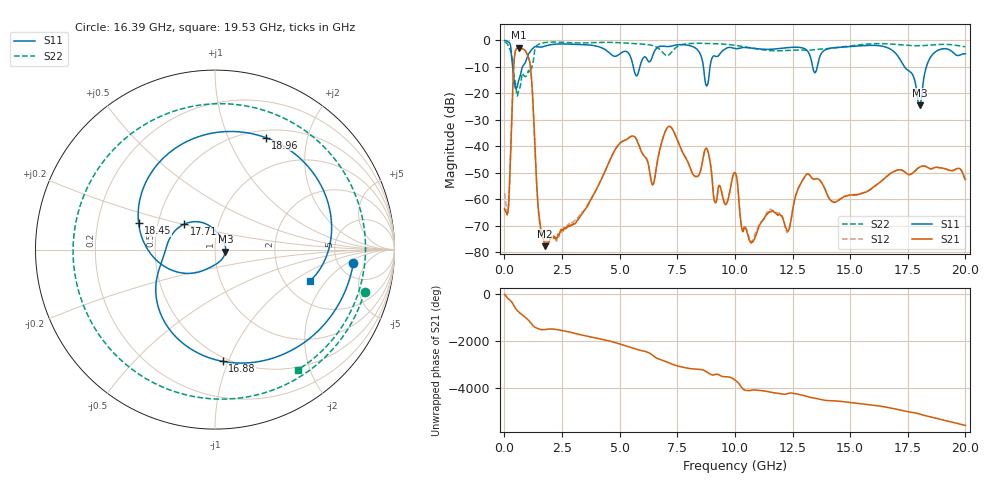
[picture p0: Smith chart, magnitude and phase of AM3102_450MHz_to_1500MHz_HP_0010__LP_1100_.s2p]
!Agilent Technologies,E8364B,MY43040894,A.07.50.67
!Agilent E8364B: A.07.50.67
!Date: Thursday, January 11, 2018 05:28:41
!Correction: S11(Full 2 Port(1,2))
!S21(Full 2 Port(1,2))
!S12(Full 2 Port(1,2))
!S22(Full 2 Port(1,2))
!S2P File: Measurements: S11, S21, S12, S22:
# Hz S  dB  R 50
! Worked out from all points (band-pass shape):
!   1601 points, 10 MHz to 20 GHz, reference 50 ohm
!   highest |S21| = -2.82 dB at 622.2 MHz (marker M1); lowest = -77.6 dB at 1.759 GHz (marker M2)
!   |S21| within 3 dB of the highest: 444.3 MHz to 1.018 GHz (573.5 MHz wide, 78.5 % of centre)
!   lowest |S11| = -24.6 dB at 18.01 GHz (marker M3), VSWR 1.13, Z = 56.2 - j1.29 ohm
!   |S11| at or under -10 dB: 356.9 MHz to 784 MHz (427.1 MHz wide, 74.9 % of centre); 5.593 GHz to 5.878 GHz (285.1 MHz wide, 4.97 % of centre); 17.35 GHz to 18.31 GHz (952.9 MHz wide, 5.34 % of centre)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
!   |S22| runs from -21.0 to -0.5 dB; largest |S21 - S12| = 0.0029
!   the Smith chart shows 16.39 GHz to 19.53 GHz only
!   S11 on the Smith chart (normalised r, x): 16.39 GHz: 6.94, -2.54; 16.88 GHz: 0.47, -0.95; 17.71 GHz: 0.68, +0.20; 18.45 GHz: 0.39, +0.14; 18.96 GHz: 0.59, +1.38; 19.53 GHz: 2.76, -1.39
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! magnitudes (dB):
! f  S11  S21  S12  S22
! 10 MHz  -0.1  -63.5  -57.6  -0.5
! 172.4 MHz  -0.6  -63.2  -63.4  -2.1
! 422.3 MHz  -15.3  -7.8  -7.8  -13.3
! 622.2 MHz  -15.1  -2.8  -2.8  -19.0
! 1.109 GHz  -4.4  -8.6  -8.6  -12.2
! 1.484 GHz  -2.5  -64.7  -65.1  -1.5
! 1.759 GHz  -2.2  -77.6  -75.8  -0.8
! 3.346 GHz  -1.6  -65.6  -65.0  -1.0
! 5.07 GHz  -4.7  -38.4  -38.4  -0.9
! 6.682 GHz  -2.5  -43.6  -43.6  -3.0
! 10.01 GHz  -3.1  -49.9  -49.8  -1.9
! 10.72 GHz  -2.9  -76.5  -75.9  -2.9
! 13.34 GHz  -8.6  -52.0  -51.9  -3.6
! 16.39 GHz  -2.2  -52.8  -53.0  -1.2
! 16.68 GHz  -3.0  -50.7  -50.7  -1.3
! 16.88 GHz  -4.1  -49.5  -49.6  -1.5
! 17.71 GHz  -13.0  -50.1  -50.1  -2.0
! 18.01 GHz  -24.6  -47.8  -47.8  -2.0
! 18.45 GHz  -6.9  -48.4  -48.4  -1.8
! 18.96 GHz  -3.3  -48.1  -48.2  -1.5
! 19.53 GHz  -5.1  -48.9  -48.8  -1.8
! 20 GHz  -5.1  -52.5  -52.6  -2.4
